|   IBIS file stm32l451_452_462_lqfp100.ibs
[IBIS ver] 4.2
[File name] stm32l451_452_462_lqfp100.ibs
[File Rev] 3.0
[Date]  05-04-2021
[Source] Data Created at STMicroelectronics
[Disclaimer]  This information is for modeling purpose only and is
   not guaranted. The information is subject to change without
   notice.
[Copyright] Copyright 2021 STMicroelectronics Inc.
|   Component stm32l451_452_462_lqfp100
[Component] stm32l451_452_462_lqfp100
[Manufacturer] STMicroelectronics
[Package]
| variable   typ   min   max
R_pkg   0.0   0.0   0.0
L_pkg   0.0H   0.0H   0.0H
C_pkg   0.0F   0.0F   0.0F
[Pin]  signal_name   model_name   R_pin   L_pin   C_pin
1 PE2 io8_ft 132.430E-3 7.034E-9 135.000E-15
2 PE3 io8_ft 133.348E-3 6.765E-9 19.500E-15
3 PE4 io8_ft 128.973E-3 6.495E-9 10.400E-15
4 PE5 io8_ft 125.345E-3 6.206E-9 5.240E-15
5 PE6-WKUP io8_ft 120.515E-3 5.991E-9 7.820E-15
6 VBAT POWER 120.471E-3 5.950E-9 6.530E-15
7 PC13 io8_ft 117.881E-3 5.783E-9 6.230E-15
8 PC14/OSC32_IN io8_ft 117.279E-3 5.654E-9 3.110E-15
9 PC15/OSC32_OUT io8_ft 115.548E-3 5.548E-9 1.390E-15
10 VSS_5 GND 114.996E-3 5.434E-9 2.920E-15
11 VDD_5 POWER 112.976E-3 5.296E-9 3.560E-15
12 PH0/OSC_IN io8_ft 111.323E-3 5.231E-9 4.780E-15
13 PH1/OSC_OUT io8_ft 109.217E-3 5.142E-9 8.660E-15
14 NRST ioreset_ft_v33 110.664E-3 5.180E-9 9.030E-15
15 PC0 io8_ft_i2c 110.608E-3 5.192E-9 7.980E-15
16 PC1 io8_ft_i2c 111.326E-3 5.252E-9 10.300E-15
17 PC2 io8_ft 114.420E-3 5.345E-9 7.000E-15
18 PC3 io8_ft 114.363E-3 5.454E-9 8.650E-15
19 VSSA_P GND 117.564E-3 5.621E-9 7.825E-15
20 VREF- GND 119.905E-3 5.800E-9 229.000E-18
21 VREF+ POWER 122.312E-3 5.963E-9 1.050E-15
22 VDDA_P POWER 125.384E-3 6.187E-9 812.000E-18
23 PA0-WKUP/CK_IN io8_ft 129.702E-3 6.485E-9 3.820E-15
24 PA1 io8_ft 132.290E-3 6.715E-9 6.800E-15
25 PA2-WKUP io8_ft 132.955E-3 7.014E-9 16.700E-15
26 PA3 io8_ft 133.943E-3 7.050E-9 17.500E-15
27 VSS_4 GND 134.958E-3 6.804E-9 12.700E-15
28 VDD_4 POWER 130.511E-3 6.528E-9 9.830E-15
29 PA4 io8_ft 125.387E-3 6.245E-9 6.070E-15
30 PA5 io8_ft 124.989E-3 6.108E-9 577.000E-18
31 PA6 io8_ft 121.784E-3 5.890E-9 1.520E-15
32 PA7 io8_ft_i2c 119.149E-3 5.716E-9 5.440E-15
33 PC4 io8_ft 116.375E-3 5.556E-9 4.100E-15
34 PC5-WKUP io8_ft 113.279E-3 5.415E-9 3.690E-15
35 PB0 io8_ft 112.727E-3 5.358E-9 3.895E-15
36 PB1 io8_ft 112.271E-3 5.272E-9 1.660E-15
37 PB2 io8_ft 111.816E-3 5.238E-9 7.920E-15
38 PE7 io8_ft 110.999E-3 5.184E-9 9.900E-15
39 PE8 io8_ft 114.589E-3 5.299E-9 7.910E-15
40 PE9 io8_ft 114.461E-3 5.333E-9 7.940E-15
41 PE10 io8_ft 115.350E-3 5.424E-9 4.180E-15
42 PE11 io8_ft 116.979E-3 5.533E-9 6.060E-15
43 PE12 io8_ft 120.185E-3 5.698E-9 5.120E-15
44 PE13 io8_ft 122.587E-3 5.871E-9 4.740E-15
45 PE14 io8_ft 126.303E-3 6.069E-9 11.600E-15
46 PE15 io8_ft 129.715E-3 6.277E-9 9.910E-15
47 PB10 io8_ft_i2c 133.373E-3 6.508E-9 5.080E-15
48 PB11 io8_ft_i2c 137.888E-3 6.857E-9 5.470E-15
49 VSSA_S GND 131.554E-3 6.802E-9 4.180E-15
50 VDD_1 POWER 132.348E-3 7.042E-9 11.900E-15
51 PB12 io8_ft 131.768E-3 7.008E-9 16.200E-15
52 PB13 io8_ft_i2c 131.784E-3 6.751E-9 2.150E-15
53 PB14 io8_ft_i2c 129.151E-3 6.483E-9 9.175E-15
54 PB15 io8_ft 125.191E-3 6.202E-9 5.663E-15
55 PD8 io8_ft 121.530E-3 5.986E-9 3.690E-15
56 PD9 io8_ft 118.874E-3 5.807E-9 7.430E-15
57 PD10 io8_ft 115.870E-3 5.635E-9 10.600E-15
58 PD11 io8_ft 113.226E-3 5.471E-9 5.760E-15
59 PD12 io8_ft_i2c 111.782E-3 5.354E-9 6.530E-15
60 PD13 io8_ft_i2c 110.713E-3 5.276E-9 11.400E-15
61 PD14 io8_ft 110.052E-3 5.204E-9 13.200E-15
62 PD15 io8_ft 109.954E-3 5.180E-9 14.600E-15
63 PC6 io8_ft 109.780E-3 5.154E-9 7.250E-15
64 PC7 io8_ft 112.446E-3 5.258E-9 359.000E-18
65 PC8 io8_ft 113.596E-3 5.332E-9 658.000E-18
66 PC9 io8_ft 115.707E-3 5.466E-9 508.500E-18
67 PA8 io8_ft 116.952E-3 5.598E-9 583.250E-18
68 PA9 io8_ft_i2c 119.043E-3 5.762E-9 545.875E-18
69 PA10 io8_ft_i2c 120.674E-3 5.880E-9 13.900E-15
70 PA11 io8_usb_lsfs_bcd_otg20_ft 124.659E-3 6.108E-9 25.000E-15
71 PA12 io8_usb_lsfs_bcd_otg20_ft 124.407E-3 6.161E-9 39.900E-15
72 PA13 io8_ft 130.156E-3 6.404E-9 302.000E-15
73 VDDUSB POWER 135.110E-3 6.824E-9 155.000E-15
74 VSS_2 GND 139.402E-3 7.077E-9 155.000E-15
75 VDD_2 POWER 133.554E-3 7.056E-9 39.000E-15
76 PA14 io8_ft 135.295E-3 7.104E-9 16.300E-15
77 PA15 io8_ft 132.514E-3 6.836E-9 9.760E-15
78 PC10 io8_ft 133.482E-3 6.641E-9 9.300E-15
79 PC11 io8_ft 128.366E-3 6.341E-9 5.420E-15
80 PC12 io8_ft 124.282E-3 6.092E-9 1.180E-15
81 PD0 io8_ft 121.841E-3 5.917E-9 5.460E-15
82 PD1 io8_ft 118.487E-3 5.728E-9 7.000E-15
83 PD2 io8_ft 117.180E-3 5.573E-9 6.060E-15
84 PD3 io8_ft 113.501E-3 5.422E-9 5.450E-15
85 PD4 io8_ft 113.789E-3 5.344E-9 529.000E-18
86 PD5 io8_ft 110.806E-3 5.256E-9 2.990E-15
87 PD6 io8_ft 110.442E-3 5.246E-9 2.060E-15
88 PD7 io8_ft 111.525E-3 5.178E-9 5.680E-15
89 PB3 io8_ft 111.144E-3 5.223E-9 9.910E-15
90 PB4 io8_ft_i2c 113.222E-3 5.310E-9 9.050E-15
91 PB5 io8_ft 113.323E-3 5.401E-9 12.900E-15
92 PB6 io8_ft_i2c 115.849E-3 5.519E-9 12.600E-15
93 PB7 io8_ft_i2c 117.578E-3 5.673E-9 6.140E-15
94 PH3/BOOT0 io8_ft 118.982E-3 5.802E-9 9.370E-15
95 PB8 io8_ft_i2c 121.886E-3 5.962E-9 7.755E-15
96 PB9 io8_ft_i2c 126.276E-3 6.158E-9 8.563E-15
97 PE0 io8_ft 128.749E-3 6.367E-9 8.159E-15
98 PE1 io8_ft 133.288E-3 6.700E-9 1.030E-15
99 EWS_BORoff GND 132.230E-3 6.844E-9 4.410E-15
100 VDD_3 POWER 132.277E-3 7.052E-9 17.100E-15
[Model Selector] io8_ft
io8_ft_ls_1v2   "GPIO - 5V tolerant - 1.2V range - Low speed"
io8_ft_ms_1v2   "GPIO - 5V tolerant - 1.2V range - Med speed"
io8_ft_fs_1v2   "GPIO - 5V tolerant - 1.2V range - Fast speed"
io8_ft_hs_1v2   "GPIO - 5V tolerant - 1.2V range - High speed"
io8_ft_ls_1v8   "GPIO - 5V tolerant - 1.8V range - Low speed"
io8_ft_ms_1v8   "GPIO - 5V tolerant - 1.8V range - Med speed"
io8_ft_fs_1v8   "GPIO - 5V tolerant - 1.8V range - Fast speed"
io8_ft_hs_1v8   "GPIO - 5V tolerant - 1.8V range - High speed"
io8_ft_ls_3v3   "GPIO - 5V tolerant - 3.3V range - Low speed"
io8_ft_ms_3v3   "GPIO - 5V tolerant - 3.3V range - Med speed"
io8_ft_fs_3v3   "GPIO - 5V tolerant - 3.3V range - Fast speed"
io8_ft_hs_3v3   "GPIO - 5V tolerant - 3.3V range - High speed"
[Model Selector] io8_ft_i2c
io8_ft_ls_1v2   "GPIO - 5V tolerant - 1.2V range - Low speed"
io8_ft_ms_1v2   "GPIO - 5V tolerant - 1.2V range - Med speed"
io8_ft_fs_1v2   "GPIO - 5V tolerant - 1.2V range - Fast speed"
io8_ft_hs_1v2   "GPIO - 5V tolerant - 1.2V range - High speed"
io8_ft_ls_1v8   "GPIO - 5V tolerant - 1.8V range - Low speed"
io8_ft_ms_1v8   "GPIO - 5V tolerant - 1.8V range - Med speed"
io8_ft_fs_1v8   "GPIO - 5V tolerant - 1.8V range - Fast speed"
io8_ft_hs_1v8   "GPIO - 5V tolerant - 1.8V range - High speed"
io8_ft_ls_3v3   "GPIO - 5V tolerant - 3.3V range - Low speed"
io8_ft_ms_3v3   "GPIO - 5V tolerant - 3.3V range - Med speed"
io8_ft_fs_3v3   "GPIO - 5V tolerant - 3.3V range - Fast speed"
io8_ft_hs_3v3   "GPIO - 5V tolerant - 3.3V range - High speed"
io8_ft_i2c_1v2   "GPIO - 5V tolerant - 1.2V range - Open drain"
io8_ft_i2c_1v8   "GPIO - 5V tolerant - 1.8V range - Open drain"
io8_ft_i2c_3v3   "GPIO - 5V tolerant - 3.3V range - Open drain"
[Model Selector] io8_usb_lsfs_bcd_otg20_ft
io8_ft_ls_1v2   "GPIO - 5V tolerant - 1.2V range - Low speed"
io8_ft_ms_1v2   "GPIO - 5V tolerant - 1.2V range - Med speed"
io8_ft_fs_1v2   "GPIO - 5V tolerant - 1.2V range - Fast speed"
io8_ft_hs_1v2   "GPIO - 5V tolerant - 1.2V range - High speed"
io8_ft_ls_1v8   "GPIO - 5V tolerant - 1.8V range - Low speed"
io8_ft_ms_1v8   "GPIO - 5V tolerant - 1.8V range - Med speed"
io8_ft_fs_1v8   "GPIO - 5V tolerant - 1.8V range - Fast speed"
io8_ft_hs_1v8   "GPIO - 5V tolerant - 1.8V range - High speed"
io8_ft_ls_3v3   "GPIO - 5V tolerant - 3.3V range - Low speed"
io8_ft_ms_3v3   "GPIO - 5V tolerant - 3.3V range - Med speed"
io8_ft_fs_3v3   "GPIO - 5V tolerant - 3.3V range - Fast speed"
io8_ft_hs_3v3   "GPIO - 5V tolerant - 3.3V range - High speed"
io8usb_ft_hs_3v3   "USB full speed"
io8usb_ft_ls_3v3   "USB low speed"
|[Model Selector] ioreset_ft_v33
|ioreset_ft_v33_1v2   "Reset PAD. 5V tolerant. 1.2V range"
|ioreset_ft_v33_1v8   "Reset PAD. 5V tolerant. 1.8V range"
|ioreset_ft_v33_3v3   "Reset PAD. 5V tolerant. 3.3V range"
[Model Selector] ioreset_ft_v33
ioreset_1v2_pu  "RESET 1.2V range with PU"
ioreset_1v2  "RESET 1.2V range"
ioreset_1v8_pu  "RESET 1.8V range with PU"
ioreset_1v8  "RESET 1.8V range"
ioreset_3v3_pu  "RESET 3.3V range with PU"
ioreset_3v3  "RESET 3.3V range"
| Models and submodels in the file (23): io8_ft_ls_1v2 (I/O), io8_ft_ms_1v2 (I/O), io8_ft_fs_1v2 (I/O), io8_ft_hs_1v2 (I/O), io8_ft_ls_1v8 (I/O), io8_ft_ms_1v8 (I/O), io8_ft_fs_1v8 (I/O), io8_ft_hs_1v8 (I/O), io8_ft_ls_3v3 (I/O), io8_ft_ms_3v3 (I/O), io8_ft_fs_3v3 (I/O), io8_ft_hs_3v3 (I/O), io8_ft_i2c_1v2 (I/O_open_drain), io8_ft_i2c_1v8 (I/O_open_drain), io8_ft_i2c_3v3 (I/O_open_drain), io8usb_ft_hs_3v3 (I/O), io8usb_ft_ls_3v3 (I/O), ioreset_1v2_pu (I/O_open_drain), ioreset_1v2 (I/O_open_drain), ioreset_1v8_pu (I/O_open_drain), ioreset_1v8 (I/O_open_drain), ioreset_3v3_pu (I/O_open_drain), ioreset_3v3 (I/O_open_drain)
